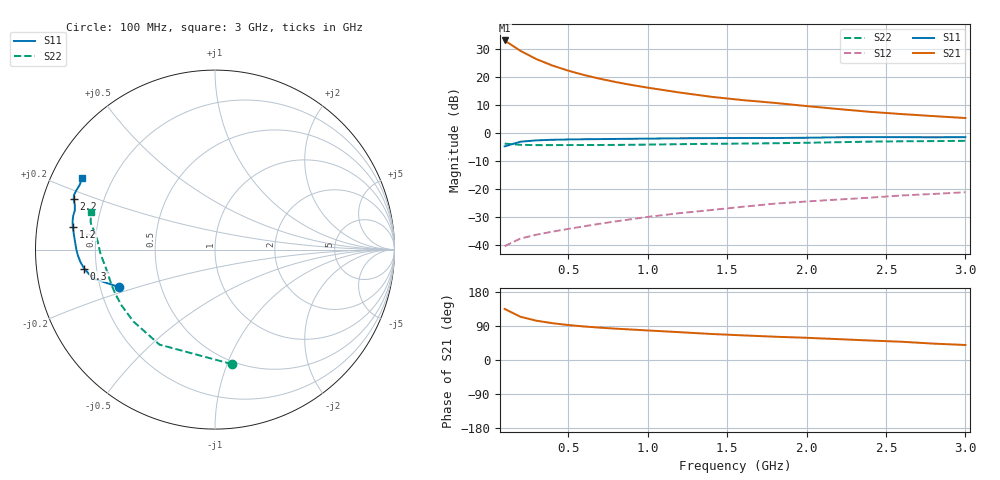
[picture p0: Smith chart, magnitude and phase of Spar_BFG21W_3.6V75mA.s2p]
! Filename: 3_675bfg21.001
! Title: BFG21W
! Bias: Vce=3.6V; Ic=75mA
! Company: NXP Semiconductors NL
! User: Quality&Reliability T&D
! Measure time: 10 Nov 1999 / 11:44:10
#  MHz  S  MA  R 50
! Freq  S11  S21  S12  S22  :
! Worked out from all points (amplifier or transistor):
!   20 points, 100 MHz to 3 GHz, reference 50 ohm
!   highest |S21| = 32.9 dB at 100 MHz (marker M1)
!   |S21| within 3 dB of that: start of sweep to 180.9 MHz
!   unconditionally stable (mu >= 1): 754.1 MHz to end of sweep
!   at 400 MHz: K = 0.81, MSG = 29.6 dB, |S12| = -35.1 dB
!   at 1.2 GHz: K = 1.07, MAG = 19.9 dB, |S12| = -28.6 dB
!   at 3 GHz: K = 1.05, MAG = 11.8 dB, |S12| = -21.1 dB
!   S11 on the Smith chart (normalised r, x): 100 MHz: 0.28, -0.17; 300 MHz: 0.15, -0.07; 1.2 GHz: 0.11, +0.08; 2.2 GHz: 0.09, +0.17; 3 GHz: 0.09, +0.25
100  0.5755 -158.8  44.17 134.8  0.009645 51.4  0.6453 -81.5
200  0.6974 -166.6  28.82 114.1  0.01321 46.6  0.6133 -120.3
300  0.7364 -171.7  20.58 103.7  0.0154 48.2  0.6059 -138.7
400  0.7542 -175.0  15.84 97.2  0.01748 51.4  0.6062 -149.0
500  0.7643 -177.5  12.82 92.3  0.01955 54.6  0.6075 -155.7
600  0.7711 -179.6  10.71 88.5  0.02178 57.5  0.6087 -160.3
700  0.7761 178.5  9.202 85.4  0.02419 60.1  0.6096 -163.9
800  0.7808 176.9  8.031 82.6  0.02665 62.1  0.6115 -166.9
900  0.7859 175.2  7.119 80.4  0.02916 64.2  0.6148 -169.5
1000  0.7913 173.7  6.389 78.0  0.032 65.6  0.6191 -171.7
1200  0.8017 171.1  5.239 73.5  0.03725 67.6  0.6298 -175.4
1400  0.8086 168.9  4.394 68.7  0.04242 68.8  0.6397 -178.4
1600  0.8122 166.7  3.831 65.0  0.04852 69.7  0.6458 179.0
1800  0.8112 164.3  3.42 61.5  0.05505 70.3  0.6545 176.2
2000  0.8198 162.3  3.004 58.6  0.06022 71.1  0.6669 173.4
2200  0.8364 160.3  2.659 55.0  0.06519 71.2  0.6828 171.0
2400  0.8426 158.5  2.369 51.4  0.07037 70.6  0.6989 169.2
2600  0.8398 156.7  2.163 48.1  0.07702 69.8  0.7094 167.6
2800  0.8356 154.4  1.99 43.2  0.082 68.2  0.7147 165.6
3000  0.8405 151.8  1.839 39.6  0.08793 67.4  0.7228 163.0
